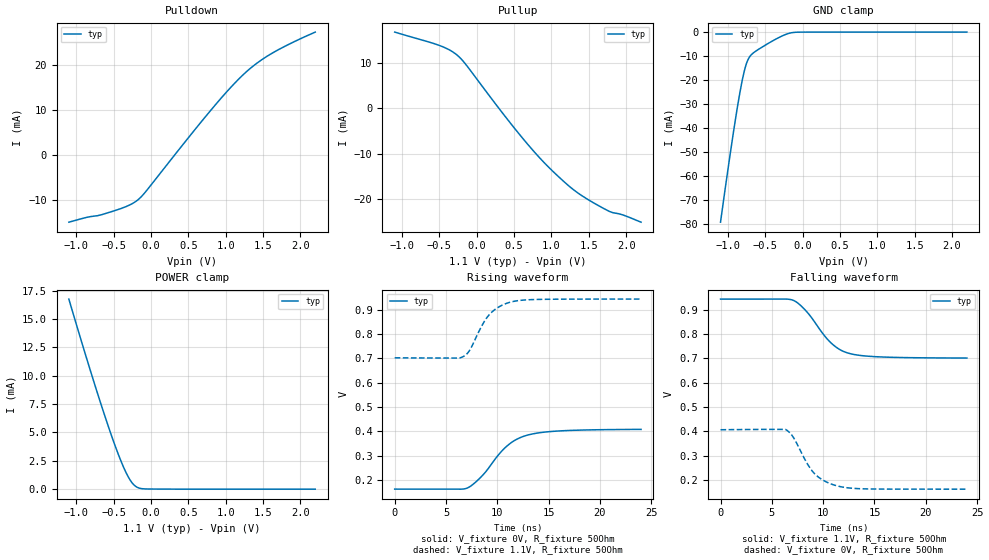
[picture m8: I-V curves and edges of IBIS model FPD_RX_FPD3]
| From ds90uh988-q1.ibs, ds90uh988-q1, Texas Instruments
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|   FPD_RX_FPD3
[Model]   FPD_RX_FPD3
Model_type   I/O
Polarity   Non-Inverting
Enable   Active-High
Vinl = 0
Vinh = 0
Vmeas = 0.55
Vref = 0.55
Cref = 0.02pF
Rref = 50
|   typ   min   max
C_comp   0.838pF   0.838pF   0.878pF
[Voltage Range]   1.1   NA   NA
[Temperature Range]   27   NA   NA
[Pullup Reference]   1.1   NA   NA
[Pulldown Reference]   -0   NA   NA
[Power Clamp Reference]   1.1   NA   NA
[GND Clamp Reference]   0   NA   NA
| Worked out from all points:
|   slope of the pulldown table from 0 to 0.165 V, typ, clamps not added: 47.5 ohm
|   slope of the pullup table from 0 to 0.165 V, typ, clamps not added: 45.2 ohm
|   GND clamp passes 1 mA (typ) near -0.23 V on its own axis
|   POWER clamp passes 1 mA (typ) near -0.30 V on its own axis
|   falling waveform, V_fixture 1.1V, R_fixture 50Ohm: 20-80 % time 2.82ns typ, NA min, NA max; typ from 0.944 V to 0.702 V
|   rising waveform, V_fixture 0V, R_fixture 50Ohm: 20-80 % time 3.15ns typ, NA min, NA max; typ from 0.162 V to 0.408 V
|   rising waveform, V_fixture 1.1V, R_fixture 50Ohm: 20-80 % time 2.08ns typ, NA min, NA max; typ from 0.703 V to 0.945 V
|   falling waveform, V_fixture 0V, R_fixture 50Ohm: 20-80 % time 2.23ns typ, NA min, NA max; typ from 0.406 V to 0.161 V
[Pulldown]
|   Voltage   I(typ)   I(min)   I(max)
-1.1V     -14.84mA   NA         NA
-661.1mV  -13.18mA   NA         NA
-506mV    -12.39mA   NA         NA
-334.4mV  -11.39mA   NA         NA
-182.6mV  -9.99mA    NA         NA
-70.4mV   -8.076mA   NA         NA
833.8mV   10.59mA    NA         NA
1.065V    14.96mA    NA         NA
1.226V    17.69mA    NA         NA
1.415V    20.33mA    NA         NA
1.629V    22.66mA    NA         NA
2.2V      27.28mA    NA         NA
[GND Clamp]
|   Voltage   I(typ)   I(min)   I(max)
-1.1V     -79.09mA   NA         NA
-977.9mV  -52.28mA   NA         NA
-925.1mV  -41.3mA    NA         NA
-875.6mV  -31.56mA   NA         NA
-812.9mV  -20.64mA   NA         NA
-779.9mV  -16.02mA   NA         NA
-746.9mV  -12.6mA    NA         NA
-710.6mV  -10.3mA    NA         NA
-657.8mV  -8.585mA   NA         NA
-275mV    -1.605mA   NA         NA
-113.3mV  -122.3uA   NA         NA
2.2V      0A         NA         NA
[Pullup]
|   Voltage   I(typ)   I(min)   I(max)
-1.1V     16.96mA    NA         NA
-509.3mV  14.05mA    NA         NA
-275mV    12.01mA    NA         NA
-136.4mV  9.552mA    NA         NA
325.6mV   -599.9uA   NA         NA
649mV     -7.304mA   NA         NA
903.1mV   -12.04mA   NA         NA
1.157V    -16.08mA   NA         NA
1.382V    -19.07mA   NA         NA
1.688V    -22.11mA   NA         NA
1.781V    -22.89mA   NA         NA
2.2V      -25.24mA   NA         NA
[POWER Clamp]
|   Voltage   I(typ)   I(min)   I(max)
-1.1V     16.75mA    NA         NA
-796.4mV  10.13mA    NA         NA
-621.5mV  6.52mA     NA         NA
-519.2mV  4.539mA    NA         NA
-400.4mV  2.453mA    NA         NA
-334.4mV  1.469mA    NA         NA
-268.4mV  698.9uA    NA         NA
-205.7mV  251.3uA    NA         NA
-136.4mV  61.72uA    NA         NA
-40.7mV   15.5uA     NA         NA
2.2V      0A         NA         NA
[Ramp]
R_load = 50
|   typ   min   max
dV/dt_r   0.147624/3.15307e-09  NA   NA
dV/dt_f   0.145684/2.81932e-09  NA   NA
[Falling Waveform]
V_fixture = 1.1V
R_fixture = 50Ohm
C_fixture = 0F
|   Time   V(typ)   V(min)   V(max)
0s        944.5mV    NA         NA
6.364ns   944.7mV    NA         NA
7.139ns   938.5mV    NA         NA
8.392ns   892.9mV    NA         NA
10.01ns   799.8mV    NA         NA
10.79ns   762.8mV    NA         NA
11.71ns   734.5mV    NA         NA
12.67ns   719.4mV    NA         NA
15.82ns   705.9mV    NA         NA
24ns      701.7mV    NA         NA
[Rising Waveform]
V_fixture = 0V
R_fixture = 50Ohm
C_fixture = 0F
|   Time   V(typ)   V(min)   V(max)
0s        161.5mV    NA         NA
7.045ns   165.6mV    NA         NA
7.61ns    180.5mV    NA         NA
8.509ns   215.8mV    NA         NA
10.16ns   305.2mV    NA         NA
11.02ns   342mV      NA         NA
12.06ns   370.4mV    NA         NA
13.22ns   386.9mV    NA         NA
16.76ns   402.7mV    NA         NA
24ns      407.5mV    NA         NA
[Rising Waveform]
V_fixture = 1.1V
R_fixture = 50Ohm
C_fixture = 0F
|   Time   V(typ)   V(min)   V(max)
0s        702.5mV    NA         NA
6.27ns    701.4mV    NA         NA
6.635ns   706.8mV    NA         NA
7.316ns   734.4mV    NA         NA
8.509ns   835.7mV    NA         NA
9.231ns   880.9mV    NA         NA
10.23ns   914mV      NA         NA
11.44ns   933.6mV    NA         NA
13.98ns   943.1mV    NA         NA
24ns      944.6mV    NA         NA
[Falling Waveform]
|Gnd
V_fixture = 0V
R_fixture = 50Ohm
C_fixture = 0F
|   Time   V(typ)   V(min)   V(max)
0s        406.3mV    NA         NA
6.353ns   407mV      NA         NA
6.69ns    396.2mV    NA         NA
7.045ns   378.3mV    NA         NA
8.392ns   270.8mV    NA         NA
9.083ns   228.9mV    NA         NA
10.09ns   196mV      NA         NA
11.44ns   174.1mV    NA         NA
14.18ns   162.6mV    NA         NA
24ns      161.5mV    NA         NA
